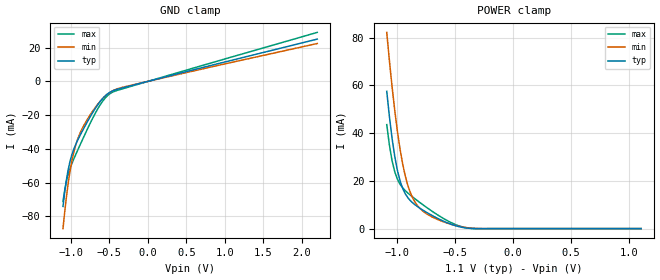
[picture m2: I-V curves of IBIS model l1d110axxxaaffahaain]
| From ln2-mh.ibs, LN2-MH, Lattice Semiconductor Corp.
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|   Model l1d110axxxaaffahaain
[Model] l1d110axxxaaffahaain
Model_type Input
Polarity   Non-Inverting
Enable   Active-High
Vinl =  0.200V
Vinh =  0.300V
C_comp   2.000pF   1.500pF   2.500pF
[Temperature Range]   25.000   0.125k   -40.000
[Voltage Range]   1.100V   1.070V   1.130V
[C Comp Corner]
C_comp   2.000pF   1.500pF   2.500pF
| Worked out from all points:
|   GND clamp passes 1 mA (typ) near -0.09 V on its own axis
|   POWER clamp passes 1 mA (typ) near -0.48 V on its own axis
[GND_clamp]
|Voltage   I(typ)   I(min)   I(max)
-1.1V     -74.11mA   -87.3mA    -71.18mA
-1.077V   -65.26mA   -77.12mA   -64.23mA
-1.054V   -57.89mA   -67.96mA   -58.93mA
-1.008V   -47.25mA   -52.99mA   -51.6mA
-962mV    -40.46mA   -42.33mA   -46.24mA
-916mV    -35.51mA   -35.04mA   -41.46mA
-847mV    -29.24mA   -27.66mA   -34.53mA
-732mV    -19.77mA   -18.77mA   -23.4mA
-617mV    -11.86mA   -11.75mA   -13.87mA
-502mV    -6.739mA   -6.846mA   -7.652mA
-272mV    -3.164mA   -2.878mA   -3.644mA
2.2V      25.09mA    22.49mA    29.07mA
[POWER_clamp]
|Voltage   I(typ)   I(min)   I(max)
-1.085V   57.54mA    82.21mA    43.56mA
-1.062V   46.9mA     70.32mA    34.95mA
-1.016V   30.2mA     49.44mA    23.76mA
-993mV    24.29mA    40.66mA    20.64mA
-947mV    16.71mA    26.8mA     17.01mA
-924mV    14.44mA    21.68mA    15.82mA
-878mV    11.52mA    14.54mA    13.85mA
-832mV    9.615mA    10.35mA    12.09mA
-763mV    7.398mA    6.902mA    9.587mA
-533mV    1.852mA    1.814mA    2.553mA
-372mV    108uA      253.3uA    136.4uA
1.1V      0A         0A         0A
